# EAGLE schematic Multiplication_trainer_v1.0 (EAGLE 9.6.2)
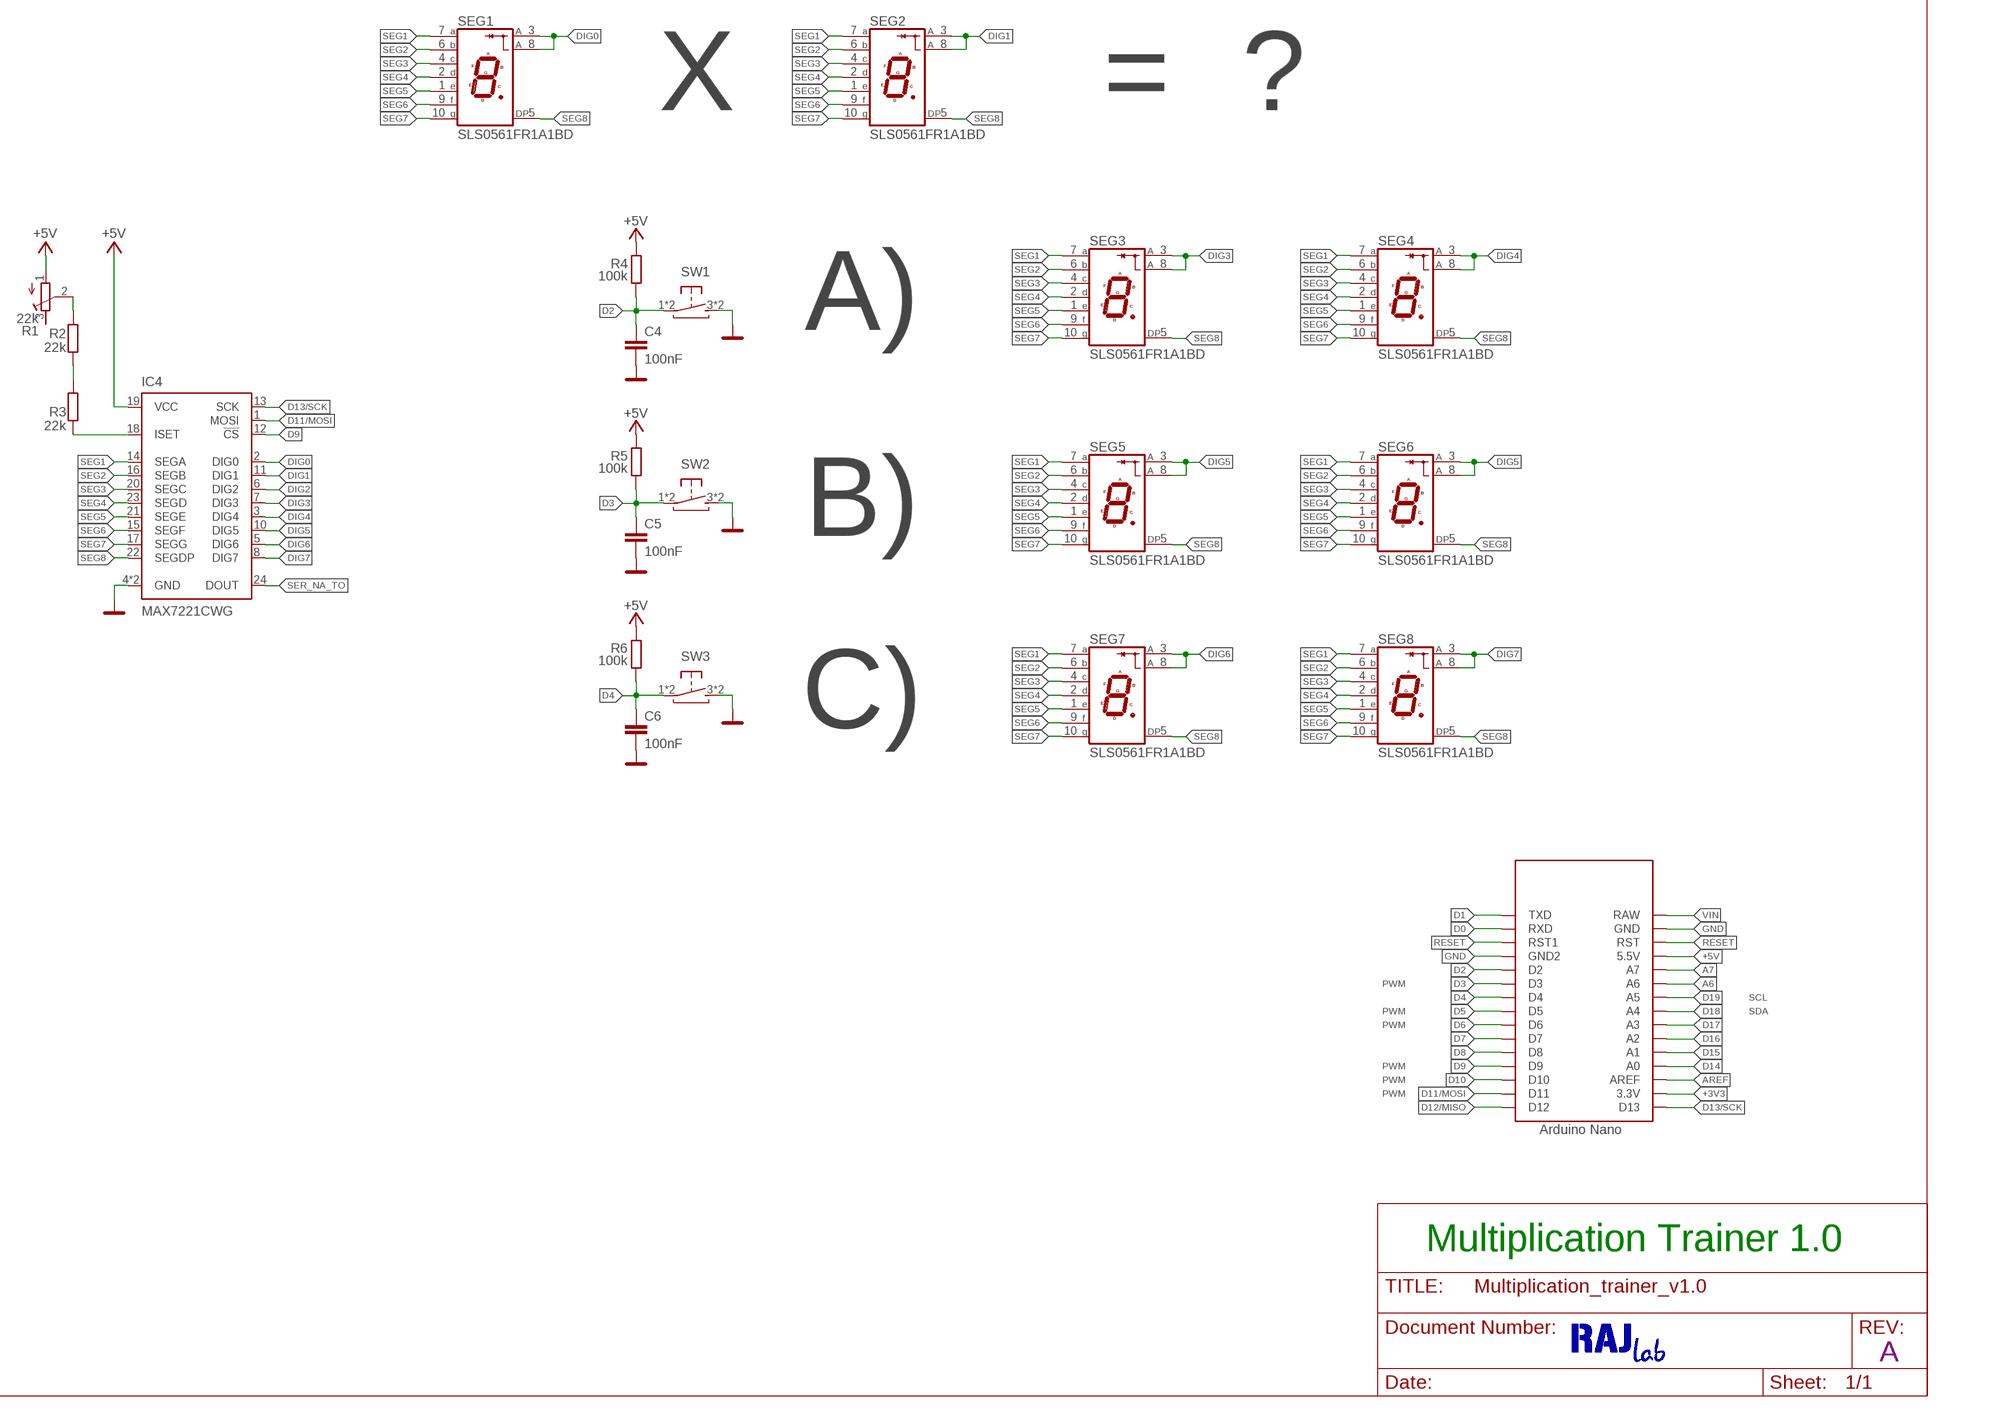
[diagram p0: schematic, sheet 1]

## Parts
C4  100nF  C-EUC0805  [C0805]
C5  100nF  C-EUC0805  [C0805]
C6  100nF  C-EUC0805  [C0805]
IC4  MAX7221CWG  [SOIC127P1032X265-24N]
R1  22k  R-TRIMM3305  [RTRIM3305]
R2  22k  R-EU_R0805  [R0805]
R3  22k  R-EU_R0805  [R0805]
R4  100k  R-EU_R0805  [R0805]
R5  100k  R-EU_R0805  [R0805]
R6  100k  R-EU_R0805  [R0805]
SEG1  SLS0561FR1A1BD  [SLS0561FR1A1BD]
SEG2  SLS0561FR1A1BD  [SLS0561FR1A1BD]
SEG3  SLS0561FR1A1BD  [SLS0561FR1A1BD]
SEG4  SLS0561FR1A1BD  [SLS0561FR1A1BD]
SEG5  SLS0561FR1A1BD  [SLS0561FR1A1BD]
SEG6  SLS0561FR1A1BD  [SLS0561FR1A1BD]
SEG7  SLS0561FR1A1BD  [SLS0561FR1A1BD]
SEG8  SLS0561FR1A1BD  [SLS0561FR1A1BD]
SW1  TACT-SW_BTNSMTJLC_6X6X4.5  [TACTSW_6X6X4.5_SMT]
SW2  TACT-SW_BTNSMTJLC_6X6X4.5  [TACTSW_6X6X4.5_SMT]
SW3  TACT-SW_BTNSMTJLC_6X6X4.5  [TACTSW_6X6X4.5_SMT]
U$2  NANOTHT-NOUSB  [NANO-NOUSB]

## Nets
+3V3: U$2.3.3V
+5V: IC4.19(VCC) R1.1(A) R4.1 R5.1 R6.1 U$2.5V(5.5V)
A6: U$2.A6
A7: U$2.A7
AREF: U$2.AREF
D0: U$2.RX1(RXD)
D1: U$2.TX0(TXD)
D2: C4.1 R4.2 SW1.1(P) SW1.2(P) U$2.D2
D3: C5.1 R5.2 SW2.1(P) SW2.2(P) U$2.D3
D4: C6.1 R6.2 SW3.1(P) SW3.2(P) U$2.D4
D5: U$2.D5
D6: U$2.D6
D7: U$2.D7
D8: U$2.D8
D9: IC4.12(!CS) U$2.D9
D10: U$2.D10
D11/MOSI: IC4.1(MOSI) U$2.D11
D12/MISO: U$2.D12
D13/SCK: IC4.13(SCK) U$2.D13
D14: U$2.A0
D15: U$2.A1
D16: U$2.A2
D17: U$2.A3
D18: U$2.A4
D19: U$2.A5
DIG0: IC4.2(DIG0) SEG1.3(CA1) SEG1.8(CA2)
DIG1: IC4.11(DIG1) SEG2.3(CA1) SEG2.8(CA2)
DIG2: IC4.6(DIG2)
DIG3: IC4.7(DIG3) SEG3.3(CA1) SEG3.8(CA2)
DIG4: IC4.3(DIG4) SEG4.3(CA1) SEG4.8(CA2)
DIG5: IC4.10(DIG5) SEG5.3(CA1) SEG5.8(CA2) SEG6.3(CA1) SEG6.8(CA2)
DIG6: IC4.5(DIG6) SEG7.3(CA1) SEG7.8(CA2)
DIG7: IC4.8(DIG7) SEG8.3(CA1) SEG8.8(CA2)
GND: C4.2 C5.2 C6.2 IC4.4(GND) IC4.9(GND) SW1.3(S) SW1.4(S) SW2.3(S) SW2.4(S) SW3.3(S) SW3.4(S) U$2.GND U$2.GND1(GND2)
N$6: IC4.18(ISET) R3.1
N$7: R2.1 R3.2
N$14: R1.2(S) R2.2
RESET: U$2.RST U$2.RST1
SEG1: IC4.14(SEGA) SEG1.7(A) SEG2.7(A) SEG3.7(A) SEG4.7(A) SEG5.7(A) SEG6.7(A) SEG7.7(A) SEG8.7(A)
SEG2: IC4.16(SEGB) SEG1.6(B) SEG2.6(B) SEG3.6(B) SEG4.6(B) SEG5.6(B) SEG6.6(B) SEG7.6(B) SEG8.6(B)
SEG3: IC4.20(SEGC) SEG1.4(C) SEG2.4(C) SEG3.4(C) SEG4.4(C) SEG5.4(C) SEG6.4(C) SEG7.4(C) SEG8.4(C)
SEG4: IC4.23(SEGD) SEG1.2(D) SEG2.2(D) SEG3.2(D) SEG4.2(D) SEG5.2(D) SEG6.2(D) SEG7.2(D) SEG8.2(D)
SEG5: IC4.21(SEGE) SEG1.1(E) SEG2.1(E) SEG3.1(E) SEG4.1(E) SEG5.1(E) SEG6.1(E) SEG7.1(E) SEG8.1(E)
SEG6: IC4.15(SEGF) SEG1.9(F) SEG2.9(F) SEG3.9(F) SEG4.9(F) SEG5.9(F) SEG6.9(F) SEG7.9(F) SEG8.9(F)
SEG7: IC4.17(SEGG) SEG1.10(G) SEG2.10(G) SEG3.10(G) SEG4.10(G) SEG5.10(G) SEG6.10(G) SEG7.10(G) SEG8.10(G)
SEG8: IC4.22(SEGDP) SEG1.5(DP) SEG2.5(DP) SEG3.5(DP) SEG4.5(DP) SEG5.5(DP) SEG6.5(DP) SEG7.5(DP) SEG8.5(DP)
SER_NA_TO: IC4.24(DOUT)
VIN: U$2.RAW
Unconnected: R1.3(E)

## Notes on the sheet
- X | = | ?
- A)
- B)
- C)
- PWM
- SCL
- PWM | SDA
- PWM
- PWM
- PWM
- PWM
- Multiplication Trainer 1.0
- A

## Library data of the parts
C4-C6 = rcl:C-EU: CAPACITOR, European symbol
IC4 = MAX7221:MAX7221CWG: 7 SEGMENT 8 DIGIT DRIVER 24SOIC Datasheet; MOUSER_NO: 710-157119S12701
R1 = rcl:R-TRIMM: Trimm resistor
R2 R3 = rcl:R-EU_: RESISTOR, European symbol; SPICEPREFIX: R
R4-R6 = resistor:R-EU_: RESISTOR, European symbol
SEG1-SEG8 = #my:SLS0561FR1A1BD; LCSC_PART: C226002
SW1-SW3 = #Ondra2:TACT-SW_BTN; LCSC_PART: C127509
U$2 = Arduino-clone:NANO: Arduino Nano

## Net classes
0 default: width 0.127 mm, drill 0.2 mm, clearance 0.127 mm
